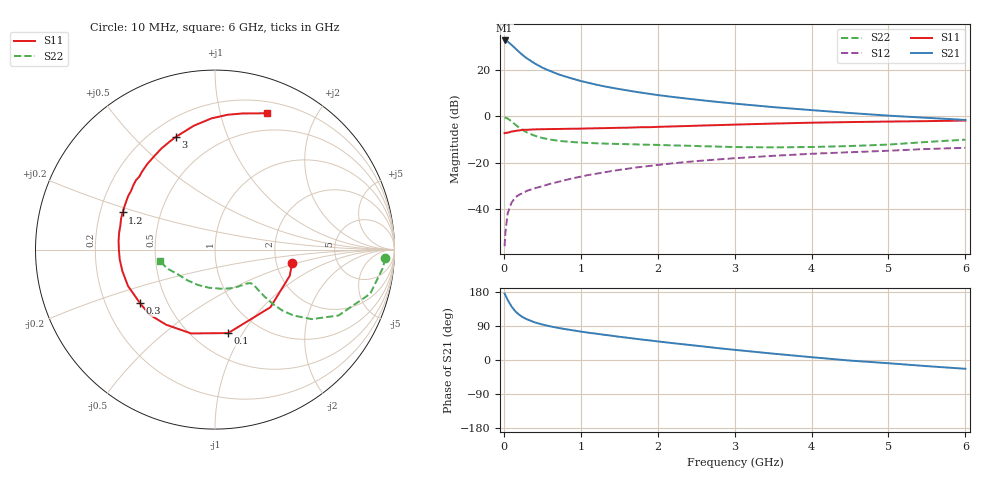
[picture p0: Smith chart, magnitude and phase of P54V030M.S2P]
! SIEMENS Small Signal Semiconductors
! BFP183
! Si NPN RF Bipolar Junction Transistor in SOT143
! VCE = 4 V  IC = 30 mA
! Common Emitter S-Parameters:  March  1996
# GHz  S  MA  R  50
!  f  S11  S21  S12  S22
! GHz  MAG  ANG  MAG  ANG  MAG  ANG  MAG  ANG
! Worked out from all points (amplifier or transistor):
!   36 points, 10 MHz to 6 GHz, reference 50 ohm
!   highest |S21| = 32.7 dB at 10 MHz (marker M1)
!   |S21| within 3 dB of that: start of sweep to 135 MHz
!   unconditionally stable (mu >= 1): 661.3 MHz to 5.675 GHz
!   at 250 MHz: K = 0.58, MSG = 29.6 dB, |S12| = -33.0 dB
!   at 1.4 GHz: K = 1.16, MAG = 15.6 dB, |S12| = -23.6 dB
!   at 6 GHz: K = 0.96, MSG = 6.0 dB, |S12| = -13.5 dB
!   S11 on the Smith chart (normalised r, x): 10 MHz: 2.45, -0.45; 100 MHz: 0.72, -0.87; 300 MHz: 0.35, -0.29; 1.2 GHz: 0.30, +0.18; 3 GHz: 0.30, +0.67; 6 GHz: 0.31, +1.41
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0.01  0.4362 -9.8  43.24 175.3  0.0016 76.2  0.9508 -2.9
0.02  0.4412 -19.4  43.22 171.2  0.0031 84.5  0.9397 -6.4
0.05  0.4455 -46.1  40.95 158.4  0.0082 77.9  0.8989 -15.9
0.1  0.4709 -81.0  34.73 141.2  0.0139 63.1  0.7796 -28.1
0.15  0.4856 -105.9  29.01 128.4  0.018 56.4  0.6637 -35.7
0.2  0.4994 -123.1  24.29 119.3  0.0206 53.2  0.5718 -40.0
0.25  0.5143 -135.4  20.55 112.5  0.0223 51.7  0.5033 -42.2
0.3  0.5135 -144.3  17.81 107.5  0.025 51.8  0.4503 -43.1
0.4  0.5255 -157.3  13.88 99.4  0.0282 52.0  0.384 -43.5
0.5  0.5297 -166.9  11.23 93.7  0.0314 53.0  0.3434 -43.2
0.6  0.5337 -174.0  9.531 88.9  0.0352 54.5  0.3173 -42.8
0.7  0.5355 -179.9  8.163 84.9  0.0386 55.5  0.2999 -42.5
0.8  0.5393 174.9  7.221 81.4  0.0424 55.9  0.2885 -42.5
1.1  0.5509 161.8  5.287 72.0  0.0547 56.9  0.2674 -44.3
1.2  0.5546 158.1  4.837 69.5  0.0582 56.8  0.264 -45.3
1.7  0.5787 142.0  3.414 56.4  0.0785 54.5  0.2498 -52.8
2.2  0.6085 128.2  2.619 44.4  0.0976 50.7  0.2372 -62.8
3  0.6652 109.0  1.887 26.8  0.1255 43.4  0.2185 -83.7
3.5  0.7003 99.7  1.586 16.8  0.1414 38.8  0.2152 -99.1
4.5  0.7547 84.6  1.183 -1.5  0.1691 29.4  0.2302 -132.1
5.5  0.7908 73.7  0.932 -16.2  0.1985 21.3  0.2816 -157.3
6  0.813 69.1  0.838 -23.2  0.2109 16.7  0.315 -168.0
